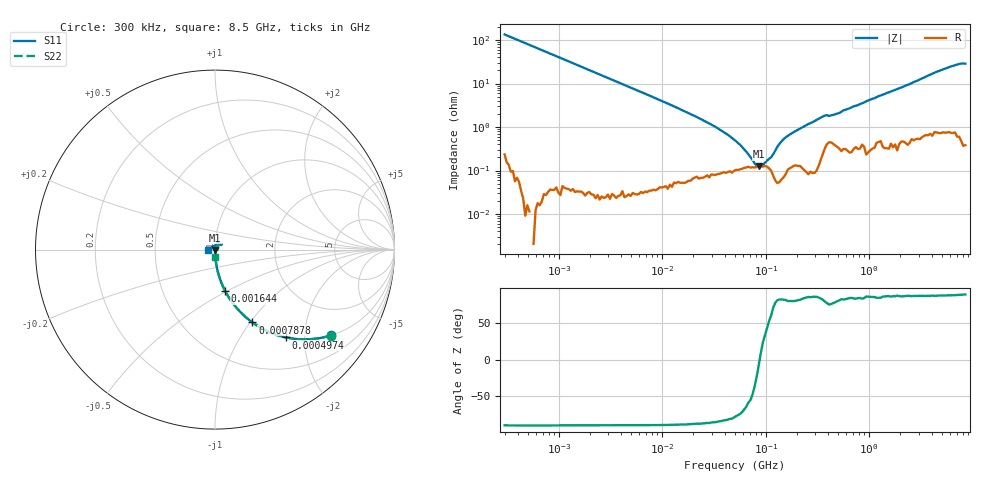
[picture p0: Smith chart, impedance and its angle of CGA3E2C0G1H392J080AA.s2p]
! S-parameter Generated by TDK Corporation
! Copyright(C) 2015 TDK Corporation.
! All Rights Reserved.
! TDK P/N: CGA3E2C0G1H392J080AA (Multilayer Ceramic Chip Capacitors)
! Property: C=3.9nF
! Size(LxWxT): 1.6x0.8x0.8mm, 0.063x0.031x0.031inches
! Model Type: s2p (Touchstone File Format Version 1.0)
! Frequency: DC=Yes Start=0.3MHz Stop=8500MHz 225points Log-sweep
! Note:
! Model Generated on Jun. 23, 2015
! Hash(MD5):
! Port Assignments:
!  1 ---| |--- 2
! Applicable Conditions:
!  Temperature = 25 degC
!  DC Bias Voltage = 0 V
!  Small Signal Operation
! Terms and conditions regarding TDK Simulation Models
! (1)This simulation model is being provided solely for informational purposes. Please refer to the specifications of the products in terms of detailed characteristics of such products.
! (2)In no event shall TDK Corporation of any of its subsidiaries be liable for any loss or damage arising, directly or indirectly,
!  From any information contained in this simulation model, including, but not limited to loss or damages arising from any inaccuracies, omissions or errors in connection with such information.
! (3)Any and all copyrights on this simulation model are owned by TDK Corporation.
!  Duplication or redistribution of this simulation model without prior written permission from TDK Corporation is prohibited.
! (4)This simulation model is subject to any modification or change without any prior notice.
! (5)Neither TDK Corporation nor any of its subsidiaries shall make any warranty, express or implied,
!  Including but not limited to the correctness, implied warranties of merchantability and fitness for a particular purpose with respect to this simulation models.
! (6)The use of this simulation model shall be deemed to have consented to the terms and conditions hereof.
# MHz S MA R 50
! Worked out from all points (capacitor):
!   224 points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, 300 kHz to 8.5 GHz, reference 50 ohm
!   read as one part in series: C = 3.94 nF near 314.1 kHz
!   lowest |Z| = 125 mohm at 85.68 MHz (marker M1)
!   series resonance near 87.47 MHz, so ESL is about 840 pH
!   S11 on the Smith chart (normalised r, x): 300 kHz: 1.00, -2.69; 497.4 kHz: 1.00, -1.62; 787.8 kHz: 1.00, -1.03; 1.644 MHz: 1.00, -0.49; 8.5 GHz: 0.92, -0.00
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0.3  0.8029 -36.6  0.5962 53.3  0.5962 53.5  0.8029 -36.6
0.4974407  0.6304 -50.9  0.7756 39.1  0.7759 39.1  0.6301 -51.0
0.7877636  0.4562 -62.8  0.8894 27.2  0.8896 27.2  0.4559 -62.8
1.643778  0.2386 -76.1  0.9709 13.8  0.9709 13.8  0.2385 -76.1
1.72111  0.2284 -76.7  0.9734 13.2  0.9733 13.2  0.2283 -76.7
9.430415  0.04216 -87.1  0.9987 2.4  0.9987 2.4  0.04229 -87.1
51.67171  0.0061 -85.9  0.9983 0.1  0.999 0.2  0.006969 -81.6
85.6787  0.002737 -83.7  0.9977 -0.2  0.9988 -0.2  0.004185 -73.4
123.7646  0.001498 -95.1  0.9985 -0.4  0.9991 -0.4  0.001976 -86.5
142.0669  0.0007741 -110.0  0.9987 -0.6  0.999 -0.5  0.0007122 -49.9
163.0757  0.0001912 137.3  0.998 -0.7  0.9987 -0.7  0.001065 -6.1
205.2186  0.001756 90.3  0.9975 -1.0  0.9982 -0.9  0.000873 -22.2
224.9819  0.002597 96.6  0.9971 -1.1  0.9981 -1.0  0.000353 -68.5
283.1228  0.003292 125.1  0.9964 -1.3  0.9971 -1.3  0.002446 112.9
356.2888  0.002902 74.2  0.9949 -1.7  0.9958 -1.7  0.006991 92.1
893.5346  0.006905 64.1  0.9951 -4.0  0.9949 -3.9  0.00312 51.9
1124.446  0.004009 73.1  0.9931 -4.9  0.9947 -5.0  0.007327 83.8
1551.304  0.007285 86.0  0.993 -6.8  0.9938 -6.7  0.008553 80.6
2456.696  0.007611 88.1  0.9922 -10.7  0.9933 -10.6  0.01177 55.5
5126.239  0.04453 46.8  0.9875 -22.3  0.9881 -22.2  0.04419 76.5
8118.083  0.02267 140.6  0.9858 -35.4  0.9867 -35.3  0.01661 -48.7
8500  0.04158 -178.6  0.9851 -37.1  0.9863 -37.1  0.04094 -88.3
